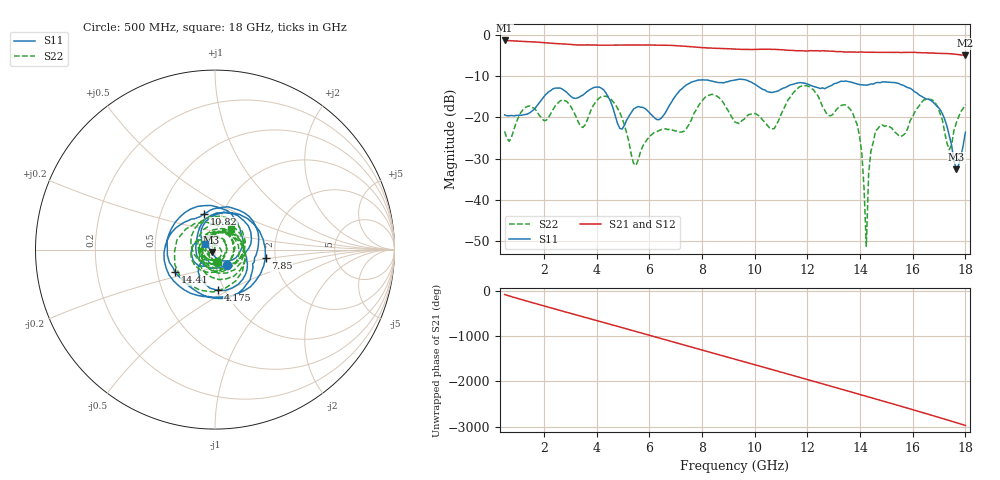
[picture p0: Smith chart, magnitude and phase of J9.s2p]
!Agilent Technologies,N5230A,MY45001360,A.07.50.67
!Agilent N5230A: A.07.50.67
!Date: Tuesday, April 16, 2024 16:05:44
!Correction: S11(Full 2 Port(1,2))
!S21(Full 2 Port(1,2))
!S12(Full 2 Port(1,2))
!S22(Full 2 Port(1,2))
!S2P File: Measurements: S11, S21, S12, S22:
# Hz S  dB  R 50
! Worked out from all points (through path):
!   201 points, 500 MHz to 18 GHz, reference 50 ohm
!   highest |S21| = -1.25 dB at 500 MHz (marker M1); lowest = -4.9 dB at 18 GHz (marker M2)
!   group delay of S21, straight-line fit = 457 ps
!   lowest |S11| = -32.6 dB at 17.65 GHz (marker M3), VSWR 1.05, Z = 48.1 - j1.34 ohm
!   |S11| at or under -10 dB: start of sweep to end of sweep
!   |S22| runs from -51.3 to -12.2 dB; largest |S21 - S12| = 0.0082
!   S11 on the Smith chart (normalised r, x): 500 MHz: 1.12, -0.19; 4.175 GHz: 0.93, -0.44; 7.85 GHz: 1.77, -0.18; 10.82 GHz: 0.82, +0.34; 14.41 GHz: 0.62, -0.17; 18 GHz: 0.89, +0.06
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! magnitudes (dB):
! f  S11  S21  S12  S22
! 500 MHz  -19.4  -1.2  -1.2  -23.4
! 2.688 GHz  -13.1  -2.1  -2.1  -15.7
! 3.475 GHz  -14.5  -2.4  -2.3  -22.4
! 4.175 GHz  -12.9  -2.4  -2.4  -14.9
! 4.875 GHz  -22.7  -2.4  -2.4  -18.8
! 5.487 GHz  -17.6  -2.3  -2.3  -31.7
! 6.362 GHz  -20.5  -2.4  -2.4  -23.2
! 7.85 GHz  -10.9  -2.9  -2.9  -17.3
! 8.463 GHz  -11.3  -3.1  -3.1  -14.5
! 9.25 GHz  -10.9  -3.4  -3.3  -21.1
! 10.82 GHz  -13.7  -3.5  -3.4  -21.7
! 12.22 GHz  -12.4  -3.8  -3.7  -13.2
! 13.89 GHz  -11.8  -4.1  -4.1  -21.7
! 14.06 GHz  -12.0  -4.0  -4.1  -28.4
! 14.24 GHz  -12.1  -4.1  -4.1  -51.3
! 14.32 GHz  -12.0  -4.1  -4.1  -33.7
! 14.41 GHz  -11.8  -4.1  -4.1  -28.2
! 15.11 GHz  -11.4  -4.2  -4.1  -22.2
! 17.04 GHz  -18.1  -4.4  -4.4  -19.0
! 17.39 GHz  -24.4  -4.5  -4.5  -27.8
! 17.65 GHz  -32.6  -4.6  -4.6  -21.4
! 18 GHz  -23.6  -4.9  -4.9  -16.9
